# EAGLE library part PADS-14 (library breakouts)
PIN HEADER
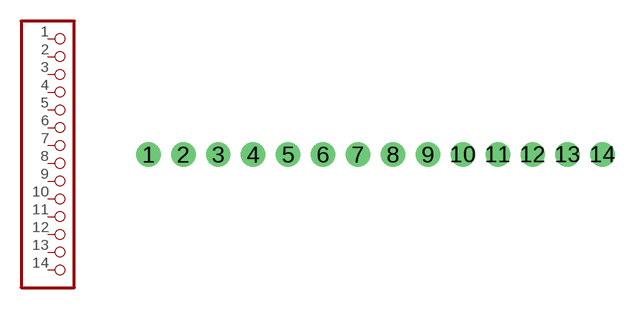
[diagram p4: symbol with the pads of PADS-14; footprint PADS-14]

Designator prefix JP

## PADS-14  [PADS-14]
1  1  pas
2  2  pas
3  3  pas
4  4  pas
5  5  pas
6  6  pas
7  7  pas
8  8  pas
9  9  pas
10  10  pas
11  11  pas
12  12  pas
13  13  pas
14  14  pas

## Footprint PADS-14 (pad centres in mm)
drill 1.016 pad 1.778: 1 -16.51,0; 2 -13.97,0; 3 -11.43,0; 4 -8.89,0; 5 -6.35,0; 6 -3.81,0; 7 -1.27,0; 8 1.27,0; 9 3.81,0; 10 6.35,0; 11 8.89,0; 12 11.43,0; 13 13.97,0; 14 16.51,0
